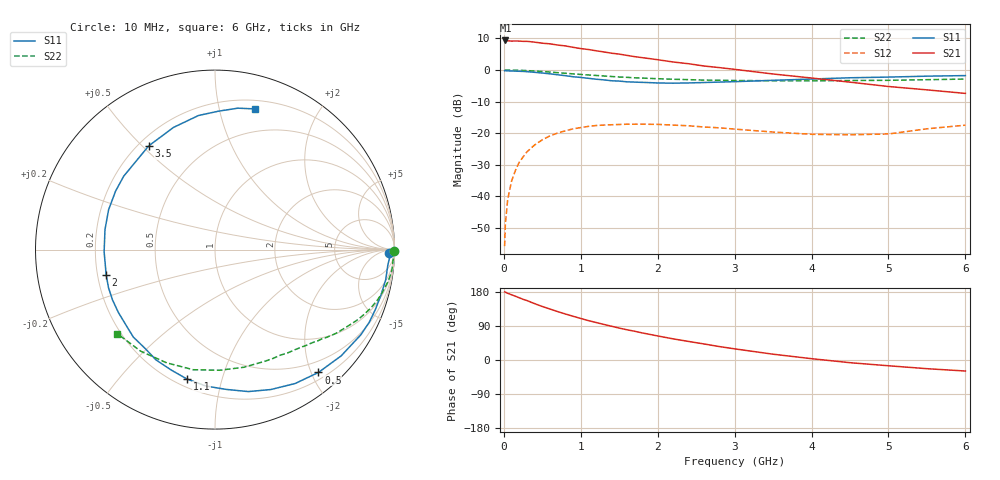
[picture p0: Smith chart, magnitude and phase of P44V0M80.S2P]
! SIEMENS Small Signal Semiconductors
! BFP182
! Si NPN RF Bipolar Junction Transistor in SOT143
! VCE = 4 V  IC = 0.8 mA
! Common Emitter S-Parameters:  March  1996
# GHz  S  MA  R  50
!  f  S11  S21  S12  S22
! GHz  MAG  ANG  MAG  ANG  MAG  ANG  MAG  ANG
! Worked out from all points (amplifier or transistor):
!   36 points, 10 MHz to 6 GHz, reference 50 ohm
!   highest |S21| = 9.4 dB at 20 MHz (marker M1)
!   |S21| within 3 dB of that: start of sweep to 1.131 GHz
!   unconditionally stable (mu >= 1): 2.782 GHz to end of sweep
!   at 250 MHz: K = 0.10, MSG = 18.3 dB, |S12| = -27.6 dB
!   at 1.4 GHz: K = 0.51, MSG = 11.4 dB, |S12| = -17.4 dB
!   at 6 GHz: K = 1.10, MAG = 3.1 dB, |S12| = -17.5 dB
!   S11 on the Smith chart (normalised r, x): 10 MHz: 51, -32; 500 MHz: 0.31, -2.11; 1.1 GHz: 0.25, -0.78; 2 GHz: 0.24, -0.11; 3.5 GHz: 0.24, +0.52; 6 GHz: 0.28, +1.29
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0.01  0.9722 -1.0  2.882 179.6  0.0016 90.3  0.9986 -0.3
0.02  0.9762 -1.9  2.943 179.0  0.0036 92.2  0.997 -0.7
0.05  0.967 -5.0  2.912 176.1  0.0088 88.7  0.9973 -1.9
0.1  0.9658 -10.0  2.872 172.2  0.0172 82.6  0.9931 -3.7
0.15  0.9589 -15.3  2.889 168.3  0.0254 79.8  0.9933 -5.6
0.3  0.9411 -30.3  2.851 156.9  0.0502 70.8  0.9782 -10.9
0.4  0.919 -40.1  2.766 148.7  0.0646 64.8  0.9622 -14.4
0.5  0.8948 -49.9  2.663 141.2  0.078 58.9  0.9465 -17.5
0.6  0.8695 -59.1  2.601 134.5  0.0902 53.2  0.9268 -20.6
0.8  0.8125 -76.8  2.411 121.4  0.1084 43.3  0.8873 -26.0
1.1  0.7378 -102.2  2.114 103.9  0.1275 30.6  0.8335 -32.7
1.3  0.697 -118.1  1.935 93.9  0.1338 23.3  0.8037 -36.6
1.5  0.6667 -133.1  1.787 84.2  0.1365 17.1  0.7742 -40.1
1.8  0.6362 -153.8  1.569 71.4  0.1383 9.8  0.7441 -44.9
2  0.6222 -167.1  1.456 63.5  0.1371 5.4  0.7275 -48.1
2.2  0.6178 -178.9  1.34 55.8  0.1335 1.8  0.7131 -51.6
2.8  0.6426 149.6  1.092 35.5  0.1209 -5.8  0.6871 -62.0
3.5  0.6858 122.6  0.864 15.3  0.1036 -7.2  0.675 -76.2
4.5  0.7528 97.0  0.641 -7.1  0.0937 3.0  0.6802 -100.3
5  0.7716 88.5  0.547 -15.2  0.0966 13.3  0.6859 -113.1
5.5  0.7982 80.8  0.484 -22.9  0.1166 16.1  0.7014 -126.3
6  0.8153 74.0  0.425 -29.1  0.1332 15.8  0.7179 -139.2
